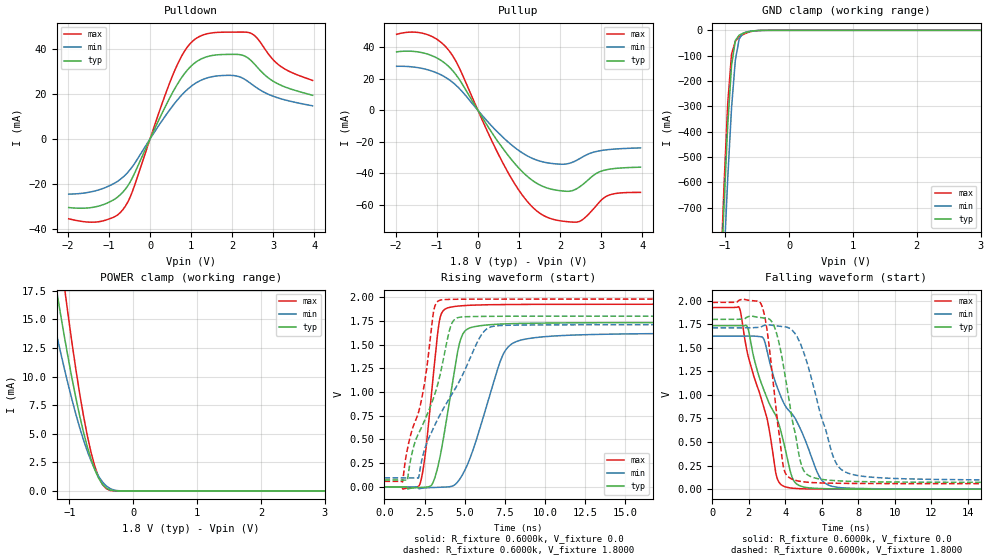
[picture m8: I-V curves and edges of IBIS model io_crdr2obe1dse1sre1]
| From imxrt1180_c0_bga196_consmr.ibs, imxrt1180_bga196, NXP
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[Model]  io_crdr2obe1dse1sre1
|   Model io_crdr2obe1dse1sre1
| This model was characterised for following simulation conditions:
| External (pad) voltage:
|   - Typ: 1.8V,   - Min: 1.71V,   - Max: 1.98V
| Library cells for typ/min/max conditions are connected as defined below:
|  PAD_IO - External Pad
|  ipp_do - Core Input
|  ipp_obe - Output Buffer Enable
|  ASRCN3V3[3] - NC
|  ASRCN3V3[4] - NC
|  ASRCP3V3[4] - NC
|  REFAPBIAS3V3 - gnde
|  REFBAMPL3V3 - vdd1v8
|  REFCAMPH3V3 - vdd1v8
|  REFDNBIAS3V3 - vdd1v8
|  REFH3V3 - REFH3V3
|  REFL3V3 - REFL3V3
|  gnde - gnde
|  ipp_dse - vdd
|  ipp_ina235_3v - NC
|  ipp_ina40_3v - NC
|  ipp_ina_mux - NC
|  ipp_ind - NC
|  ipp_ind_1p8v - NC
|  ipp_ind_3v - NC
|  ipp_sre - vdd
|  vdd - vdd
|  vdd1v8 - vdd1v8
|  vdda - vdde3v3
|  vdde3v3 - vdde3v3
| All other pins connected to ground
Model_type I/O
Polarity   Non-Inverting
Enable   Active-High
Vinl =   0.5400V
Vinh =   1.2600V
Vmeas =  0.9000V
Cref =   15.0000pF
Rref =   0.6000k
Vref =   0.0V
C_comp   3.9792pF   3.7942pF   4.1043pF
|C_comp_pullup   0.4868pF   0.5823pF   0.4755pF
|C_comp_pulldown   2.0822pF   2.1674pF   1.8518pF
[Model Spec]
| variable   typ   min   max
Vinh   1.2600V   NA   NA
Vinl   0.5400V   NA   NA
Vref   0.0V   0.0V   0.0V
Cref   15.0000pF   15.0000pF   15.0000pF
Rref   0.6000k   0.6000k   0.6000k
[Receiver Thresholds]
Vcross_high  =   0.0V
Vcross_low  =   0.0V
Vdiff_ac  =   0.0V
Vdiff_dc  =   0.0V
Tdiffslew_ac  =   0.0S
[Temperature Range]   25.0000   0.1250k   -40.0000
[Voltage Range]   1.8000V   1.7100V   1.9800V
[Pullup Reference]   1.8000V   1.7100V   1.9800V
[Pulldown Reference]   0.0V   0.0V   0.0V
[POWER Clamp Reference]   1.8000V   1.7100V   1.9800V
[GND Clamp Reference]   0.0V   0.0V   0.0V
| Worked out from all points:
|   slope of the pulldown table from 0 to 0.27 V, typ, clamps not added: 25.6 ohm
|   slope of the pullup table from 0 to 0.27 V, typ, clamps not added: 23.8 ohm
|   GND clamp passes 1 mA (typ) near -0.50 V on its own axis
|   POWER clamp passes 1 mA (typ) near -0.53 V on its own axis
|   rising waveform, R_fixture 0.6000k, V_fixture 0.0: 20-80 % time 1.02ns typ, 1.79ns min, 692ps max; typ from 0 V to 1.73 V
|   rising waveform, R_fixture 0.6000k, V_fixture 1.8000: 20-80 % time 1.99ns typ, 2.88ns min, 1.39ns max; typ from 0.072 V to 1.8 V
|   falling waveform, R_fixture 0.6000k, V_fixture 0.0: 20-80 % time 1.8ns typ, 2.26ns min, 1.49ns max; typ from 1.73 V to 0 V
|   falling waveform, R_fixture 0.6000k, V_fixture 1.8000: 20-80 % time 937ps typ, 1.38ns min, 686ps max; typ from 1.8 V to 0.072 V
[Pulldown]
|Voltage   I(typ)   I(min)   I(max)
-1.98V    -30.4mA    -24.44mA   -35.4mA
-1.2V     -29.48mA   -22.28mA   -36.54mA
-840mV    -26.45mA   -19.34mA   -34.25mA
-600mV    -22.26mA   -15.94mA   -29.79mA
-420mV    -16.87mA   -12.03mA   -22.87mA
600mV     22.22mA    15.79mA    30.28mA
900mV     30.36mA    21.79mA    40.52mA
1.14V     34.38mA    25.06mA    44.79mA
1.98V     37.51mA    28.2mA     47.38mA
2.46V     34.79mA    24.52mA    46.85mA
3.12V     24.4mA     18.2mA     33.06mA
3.96V     19.37mA    14.7mA     25.97mA
[Pullup]
|Voltage   I(typ)   I(min)   I(max)
-1.98V    37.17mA    27.99mA    48.3mA
-1.26V    36mA       26.04mA    48.37mA
-720mV    28.06mA    19.81mA    38.46mA
-480mV    20.65mA    14.61mA    28.37mA
240mV     -10.13mA   -7.213mA   -13.9mA
720mV     -28.1mA    -19.75mA   -38.89mA
1.14V     -40.44mA   -27.98mA   -55.87mA
1.56V     -48.07mA   -32.59mA   -66.23mA
2.16V     -51.42mA   -34.03mA   -70.68mA
2.46V     -48.9mA    -30.94mA   -70.69mA
3.12V     -37.78mA   -25.09mA   -54.69mA
3.96V     -36.1mA    -23.86mA   -52.12mA
[GND_clamp]
|Voltage   I(typ)   I(min)   I(max)
-1.98V    -7.543A    -7.6A      -7.897A
-1.08V    -1.077A    -1.286A    -1.025A
-1.02V    -705.3mA   -921.3mA   -628.8mA
-960mV    -377.1mA   -587.4mA   -291.7mA
-900mV    -139.2mA   -307mA     -94.38mA
-840mV    -40.12mA   -117mA     -42.82mA
-780mV    -18.81mA   -33.95mA   -26.13mA
-720mV    -11.86mA   -11.44mA   -16.78mA
-660mV    -7.061mA   -5.737mA   -9.992mA
-540mV    -1.684mA   -1.901mA   -2.15mA
-420mV    -207.1uA   -403.7uA   -160.6uA
3.96V     0A         0A         0A
[POWER_clamp]
|Voltage   I(typ)   I(min)   I(max)
-1.98V    46.79mA    35.94mA    61.38mA
-1.32V    21.77mA    16.85mA    28.91mA
-1.2V     17.57mA    13.71mA    23.33mA
-1.14V    15.55mA    12.2mA     20.62mA
-1.08V    13.59mA    10.75mA    17.99mA
-1.02V    11.7mA     9.353mA    15.46mA
-900mV    8.209mA    6.76mA     10.73mA
-720mV    3.898mA    3.51mA     4.887mA
-540mV    1.103mA    1.267mA    1.195mA
-420mV    244.5uA    429.2uA    190.6uA
-180mV    280.9nA    5.273uA    26.8nA
3.96V     0A         0A         0A
[Ramp]
| variable   typ   min   max
dV/dt_r  1.0396/1.0213n   0.9730/1.7873n   1.1554/0.6921n
dV/dt_f  1.0366/0.9367n   0.9689/1.3831n   1.1528/0.6862n
R_load = 0.6000k
[Rising Waveform]
R_fixture= 0.6000k
V_fixture= 0.0
V_fixture_min= 0.0
V_fixture_max= 0.0
|time   V(typ)   V(min)   V(max)
0s        47.1nV     1.315uV    17.96nV
2.2ns     -7.252mV   -18.71mV   23.33mV
2.558ns   -3.205mV   -10.3mV    357.3mV
3.429ns   284.5mV    -4.515mV   1.748V
4.151ns   1.002V     4.225mV    1.896V
4.634ns   1.481V     67.01mV    1.907V
5.072ns   1.651V     195.1mV    1.912V
7.398ns   1.718V     1.394V     1.922V
8.855ns   1.725V     1.56V      1.924V
60ns      1.733V     1.622V     1.926V
[Rising Waveform]
R_fixture= 0.6000k
V_fixture= 1.8000
V_fixture_min= 1.7100
V_fixture_max= 1.9800
|time   V(typ)   V(min)   V(max)
0s        72.29mV    95.11mV    58.66mV
1.134ns   71.85mV    95.04mV    53.5mV
1.431ns   69.61mV    94.71mV    399.4mV
2.122ns   560.5mV    94.2mV     783.7mV
3.075ns   942.8mV    626mV      1.856V
3.54ns    1.234V     783.8mV    1.971V
4.358ns   1.762V     1.018V     1.978V
6.038ns   1.797V     1.601V     1.979V
6.991ns   1.798V     1.698V     1.98V
60ns      1.8V       1.71V      1.98V
[Falling Waveform]
R_fixture= 0.6000k
V_fixture= 0.0
V_fixture_min= 0.0
V_fixture_max= 0.0
|time   V(typ)   V(min)   V(max)
0s        1.733V     1.622V     1.926V
1.453ns   1.734V     1.622V     1.931V
1.911ns   1.723V     1.621V     1.452V
2.793ns   1.066V     1.6V       887mV
3.541ns   749mV      1.087V     120.4mV
4.231ns   217.7mV    824mV      14.02mV
4.647ns   50.3mV     710mV      6.342mV
5.932ns   6.268mV    111mV      1.147mV
7.044ns   2.628mV    15.53mV    367.3uV
60ns      2.987uV    6.213uV    1.309uV
[Falling Waveform]
R_fixture= 0.6000k
V_fixture= 1.8000
V_fixture_min= 1.7100
V_fixture_max= 1.9800
|time   V(typ)   V(min)   V(max)
0s        1.8V       1.71V      1.98V
2.665ns   1.819V     1.72V      1.965V
2.966ns   1.813V     1.741V     1.729V
3.365ns   1.738V     1.735V     1.069V
3.904ns   1.297V     1.724V     225.6mV
4.788ns   322.4mV    1.559V     83.29mV
5.269ns   145.1mV    1.287V     72.6mV
6.706ns   90.22mV    304.6mV    62.68mV
8.184ns   79.83mV    137.8mV    60.09mV
60ns      72.29mV    95.12mV    58.66mV
